| This Model is valid for Automotive grade 2 Temperature Range -40C<=Tc<=105C
| Valid for LPDDR4-4266 operation
| Part Number   VDD/VDDQ   Package   Architecture
| SCE11U48324AF-04ZA2   1.1 +0.07/-0.04  FBGA   1.5G bit x 32 (200b,QDP,10x14.5x1.1)
[IBIS Ver]  5.0
[File Name] usesnxx32aa2.ibs
[Date]   06/26/2025
[File Rev]  1.0
[Source] Simulation of a silicon level SPICE model
[Notes]  IBIS Characteristics for I/O Buffer
  IBIS Model Revision History: Rev 1.0:
  2025-06-26 - IBIS model file initial creation
[Disclaimer]  The IBIS models are for modeling purpose only and are subject to change without any notice. UniIC is not
  responsible for any problems the models may cause.
[Copyright] Copyright 2025 UniIC Semiconductors Corp. All rights reserved
|   Component SCE11U48324AF-04ZA2
[Component] SCE11U48324AF-04ZA2
[Manufacturer] UniIC Semiconductors Corp.
[Package]
|   typ   min   max
R_pkg   1377.8m   678.01m   2200.4m
L_pkg   2.871nH   1.351nH   4.718nH
C_pkg   1.060pF   0.653pF   1.525pF
[Pin] signal_name  model_name   R_pin   L_pin   C_pin
A1   DNU   NC
A2   DNU   NC
A3   VSS   GND
A4   VDD2   POWER
A5   ZQ0   NC
A8   ZQ1   NC
A9   VDD2   POWER
A10   VSS   GND
A11   DNU   NC
A12   DNU   NC
B1   DNU   NC
B2   DQ0_A   DQ   815.75m   1.783nH   0.708pF
B3   VDDQ   POWER
B4   DQ7_A   DQ   837.92m   1.787nH   0.739pF
B5   VDDQ   POWER
B8   VDDQ   POWER
B9   DQ15_A   DQ   841.56m   1.773nH   0.739pF
B10   VDDQ   POWER
B11   DQ8_A   DQ   884.91m   1.894nH   0.764pF
B12   DNU   NC
C1   VSS   GND
C2   DQ1_A   DQ   862.48m   1.799nH   0.724pF
C3   DMI0_A   DQ   832.58m   1.719nH   0.717pF
C4   DQ6_A   DQ   753.90m   1.588nH   0.689pF
C5   VSS   GND
C8   VSS   GND
C9   DQ14_A   DQ   814.61m   1.676nH   0.743pF
C10   DMI1_A   DQ   820.28m   1.690nH   0.736pF
C11   DQ9_A   DQ   853.94m   1.774nH   0.747pF
C12   VSS   GND
D1   VDDQ   POWER
D2   VSS   GND
D3   DQS0_t_A   DQS   780.62m   1.630nH   0.669pF
D4   VSS   GND
D5   VDDQ   POWER
D8   VDDQ   POWER
D9   VSS   GND
D10   DQS1_t_A   DQS   780.55m   1.628nH   0.668pF
D11   VSS   GND
D12   VDDQ   POWER
E1   VSS   GND
E2   DQ2_A   DQ   769.99m   1.582nH   0.719pF
E3   DQS0_c_A   DQS   796.22m   1.643nH   0.667pF
E4   DQ5_A   DQ   693.55m   1.405nH   0.687pF
E5   VSS   GND
E8   VSS   GND
E9   DQ13_A   DQ   692.33m   1.403nH   0.695pF
E10   DQS1_c_A   DQS   796.67m   1.642nH   0.671pF
E11   DQ10_A   DQ   751.10m   1.558nH   0.707pF
E12   VSS   GND
F1   VDD1   POWER
F2   DQ3_A   DQ   803.96m   1.656nH   0.728pF
F3   VDDQ   POWER
F4   DQ4_A   DQ   678.01m   1.373nH   0.653pF
F5   VDD2   POWER
F8   VDD2   POWER
F9   DQ12_A   DQ   678.86m   1.351nH   0.678pF
F10   VDDQ   POWER
F11   DQ11_A   DQ   777.70m   1.621nH   0.719pF
F12   VDD1   POWER
G1   VSS   GND
G2   NC   NC
G3   VSS   GND
G4   VDD1   POWER
G5   VSS   GND
G8   VSS   GND
G9   VDD1   POWER
G10   VSS   GND
G11   NC   NC
G12   VSS   GND
H1   VDD2   POWER
H2   CA0_A   CA_INPUT   1149.9m   2.416nH   0.957pF
H3   CS1_A   CS_INPUT
H4   CS0_A   CS_INPUT
H5   VDD2   POWER
H8   VDD2   POWER
H9   CA2_A   CA_INPUT   1114.3m   2.201nH   0.964pF
H10   CA3_A   CA_INPUT   1179.0m   2.324nH   1.007pF
H11   CA4_A   CA_INPUT   1281.5m   2.502nH   1.076pF
H12   VDD2   POWER
J1   VSS   GND
J2   CA1_A   CA_INPUT   1241.5m   2.547nH   1.026pF
J3   VSS   GND
J4   CKE0_A   CKE_INPUT
J5   CKE1_A   CKE_INPUT
J8   CK_t_A   CLK_INPUT   1164.4m   2.511nH   0.936pF
J9   CK_c_A   CLK_INPUT   1179.6m   2.532nH   0.945pF
J10   VSS   GND
J11   CA5_A   CA_INPUT   1353.8m   2.632nH   1.108pF
J12   VSS   GND
K1   VDD2   POWER
K2   VSS   GND
K3   VDD2   POWER
K4   VSS   GND
K5   NC   NC
K8   NC   NC
K9   VSS   GND
K10   VDD2   POWER
K11   VSS   GND
K12   VDD2   POWER
N1   VDD2   POWER
N2   VSS   GND
N3   VDD2   POWER
N4   VSS   GND
N5   NC   NC
N8   NC   NC
N9   VSS   GND
N10   VDD2   POWER
N11   VSS   GND
N12   VDD2   POWER
P1   VSS   GND
P2   CA1_B   CA_INPUT   1537.5m   3.379nH   1.134pF
P3   VSS   GND
P4   CKE0_B   CKE_INPUT
P5   CKE1_B   CKE_INPUT
P8   CK_t_B   CLK_INPUT   1530.3m   3.244nH   1.121pF
P9   CK_c_B   CLK_INPUT   1598.7m   3.371nH   1.166pF
P10   VSS   GND
P11   CA5_B   CA_INPUT   1748.8m   3.785nH   1.229pF
P12   VSS   GND
R1   VDD2   POWER
R2   CA0_B   CA_INPUT   1568.1m   3.442nH   1.146pF
R3   CS1_B   CS_INPUT
R4   CS0_B   CS_INPUT
R5   VDD2   POWER
R8   VDD2   POWER
R9   CA2_B   CA_INPUT   1529.7m   3.316nH   1.089pF
R10   CA3_B   CA_INPUT   1595.3m   3.372nH   1.142pF
R11   CA4_B   CA_INPUT   1737.9m   3.619nH   1.236pF
R12   VDD2   POWER
T1   VSS   GND
T2   NC   NC
T3   VSS   GND
T4   VDD1   POWER
T5   VSS   GND
T8   VSS   GND
T9   VDD1   POWER
T10   VSS   GND
T11   RESET_n   NC
T12   VSS   GND
U1   VDD1   POWER
U2   DQ3_B   DQ   1783.2m   3.716nH   1.313pF
U3   VDDQ   POWER
U4   DQ4_B   DQ   1690.1m   3.453nH   1.244pF
U5   VDD2   POWER
U8   VDD2   POWER
U9   DQ12_B   DQ   1997.2m   3.951nH   1.469pF
U10   VDDQ   POWER
U11   DQ11_B   DQ   2089.2m   4.305nH   1.506pF
U12   VDD1   POWER
V1   VSS   GND
V2   DQ2_B   DQ   1862.6m   3.936nH   1.329pF
V3   DQS0_c_B   DQS   1877.9m   4.033nH   1.335pF
V4   DQ5_B   DQ   1694.8m   3.459nH   1.250pF
V5   VSS   GND
V8   VSS   GND
V9   DQ13_B   DQ   1972.8m   3.803nH   1.473pF
V10   DQS1_c_B   DQS   2092.9m   4.378nH   1.478pF
V11   DQ10_B   DQ   2200.4m   4.718nH   1.525pF
V12   VSS   GND
W1   VDDQ   POWER
W2   VSS   GND
W3   DQS0_t_B   DQS   1860.3m   4.071nH   1.335pF
W4   VSS   GND
W5   VDDQ   POWER
W8   VDDQ   POWER
W9   VSS   GND
W10   DQS1_t_B   DQS   2120.7m   4.481nH   1.515pF
W11   VSS   GND
W12   VDDQ   POWER
Y1   VSS   GND
Y2   DQ1_B   DQ   2023.5m   4.328nH   1.424pF
Y3   DMI0_B   DQ   1786.4m   3.621nH   1.340pF
Y4   DQ6_B   DQ   1702.5m   3.534nH   1.251pF
Y5   VSS   GND
Y8   VSS   GND
Y9   DQ14_B   DQ   1982.9m   3.898nH   1.426pF
Y10   DMI1_B   DQ   2061.8m   4.157nH   1.462pF
Y11   DQ9_B   DQ   2177.0m   4.685nH   1.515pF
Y12   VSS   GND
AA1   DNU   NC
AA2   DQ0_B   DQ   2060.0m   4.290nH   1.449pF
AA3   VDDQ   POWER
AA4   DQ7_B   DQ   1733.2m   3.601nH   1.258pF
AA5   VDDQ   POWER
AA8   VDDQ   POWER
AA9   DQ15_B   DQ   1970.9m   3.988nH   1.397pF
AA10  VDDQ   POWER
AA11  DQ8_B   DQ   2099.3m   4.696nH   1.451pF
AA12  DNU   NC
AB1   DNU   NC
AB2   DNU   NC
AB3   VSS   GND
AB4   VDD2   POWER
AB5   VSS   GND
AB8   VSS   GND
AB9   VDD2   POWER
AB10  VSS   GND
AB11  DNU   NC
AB12  DNU   NC
[Diff Pin]  inv_pin  vdiff   tdelay_typ   tdelay_min   tdelay_max
D3   E3   0.120V   0.000s   NA   NA
W3   V3   0.120V   0.000s   NA   NA
D10   E10   0.120V   0.000s   NA   NA
W10   V10   0.120V   0.000s   NA   NA
J8   J9   0.145V   0.000s   NA   NA
P8   P9   0.145V   0.000s   NA   NA
|   Model Selector
[Model Selector] DQ
| Data I/O models
DQ_PD40_SOC-ODT40_VOH30_4266   40 Ohm Pulldown, 40 Ohm System ODT Setting, VOH=VDDQ/3.0, 3200-4266Mbps
DQ_PD40_SOC-ODT48_VOH30_4266   40 Ohm Pulldown, 48 Ohm System ODT Setting, VOH=VDDQ/3.0, 3200-4266Mbps
DQ_PD40_SOC-ODT60_VOH30_4266   40 Ohm Pulldown, 60 Ohm System ODT Setting, VOH=VDDQ/3.0, 3200-4266Mbps
DQ_PD40_SOC-ODT80_VOH30_4266   40 Ohm Pulldown, 80 Ohm System ODT Setting, VOH=VDDQ/3.0, 3200-4266Mbps
DQ_PD40_SOC-ODT120_VOH30_4266   40 Ohm Pulldown, 120 Ohm System ODT Setting, VOH=VDDQ/3.0, 3200-4266Mbps
DQ_PD40_SOC-ODT240_VOH30_4266   40 Ohm Pulldown, 240 Ohm System ODT Setting, VOH=VDDQ/3.0, 3200-4266Mbps
DQ_PD40_SOC-ODTDIS_VOH30_4266   40 Ohm Pulldown, SOC ODT disabled setting, VOH=VDDQ/3.0 cal. point, 3200-4266Mbps
DQ_PD40_SOC-ODT80_VOH25_4266   40 Ohm Pulldown, 80 Ohm System ODT Setting, VOH=VDDQ/2.5, 3200-4266Mbps
DQ_PD40_SOC-ODT120_VOH25_4266   40 Ohm Pulldown, 120 Ohm System ODT Setting, VOH=VDDQ/2.5, 3200-4266Mbps
DQ_PD40_SOC-ODT240_VOH25_4266   40 Ohm Pulldown, 240 Ohm System ODT Setting, VOH=VDDQ/2.5, 3200-4266Mbps
DQ_PD40_SOC-ODTDIS_VOH25_4266   40 Ohm Pulldown, SOC ODT disabled setting, VOH=VDDQ/2.5 cal. point, 3200-4266Mbps
DQ_PD48_SOC-ODT40_VOH30_4266   48 Ohm Pulldown, 40 Ohm System ODT Setting, VOH=VDDQ/3.0, 3200-4266Mbps
DQ_PD48_SOC-ODT48_VOH30_4266   48 Ohm Pulldown, 48 Ohm System ODT Setting, VOH=VDDQ/3.0, 3200-4266Mbps
DQ_PD48_SOC-ODT60_VOH30_4266   48 Ohm Pulldown, 60 Ohm System ODT Setting, VOH=VDDQ/3.0, 3200-4266Mbps
DQ_PD48_SOC-ODT80_VOH30_4266   48 Ohm Pulldown, 80 Ohm System ODT Setting, VOH=VDDQ/3.0, 3200-4266Mbps
DQ_PD48_SOC-ODT120_VOH30_4266   48 Ohm Pulldown, 120 Ohm System ODT Setting, VOH=VDDQ/3.0, 3200-4266Mbps
DQ_PD48_SOC-ODT240_VOH30_4266   48 Ohm Pulldown, 240 Ohm System ODT Setting, VOH=VDDQ/3.0, 3200-4266Mbps
DQ_PD48_SOC-ODTDIS_VOH30_4266   48 Ohm Pulldown, SOC ODT disabled setting, VOH=VDDQ/3.0 cal. point, 3200-4266Mbps
DQ_PD48_SOC-ODT80_VOH25_4266   48 Ohm Pulldown, 80 Ohm System ODT Setting, VOH=VDDQ/2.5, 3200-4266Mbps
DQ_PD48_SOC-ODT120_VOH25_4266   48 Ohm Pulldown, 120 Ohm System ODT Setting, VOH=VDDQ/2.5, 3200-4266Mbps
DQ_PD48_SOC-ODT240_VOH25_4266   48 Ohm Pulldown, 240 Ohm System ODT Setting, VOH=VDDQ/2.5, 3200-4266Mbps
DQ_PD48_SOC-ODTDIS_VOH25_4266   48 Ohm Pulldown, SOC ODT disabled setting, VOH=VDDQ/2.5 cal. point, 3200-4266Mbps
DQ_PD60_SOC-ODT40_VOH30_4266   60 Ohm Pulldown, 40 Ohm System ODT Setting, VOH=VDDQ/3.0, 3200-4266Mbps
DQ_PD60_SOC-ODT48_VOH30_4266   60 Ohm Pulldown, 48 Ohm System ODT Setting, VOH=VDDQ/3.0, 3200-4266Mbps
DQ_PD60_SOC-ODT60_VOH30_4266   60 Ohm Pulldown, 60 Ohm System ODT Setting, VOH=VDDQ/3.0, 3200-4266Mbps
DQ_PD60_SOC-ODT80_VOH30_4266   60 Ohm Pulldown, 80 Ohm System ODT Setting, VOH=VDDQ/3.0, 3200-4266Mbps
DQ_PD60_SOC-ODT120_VOH30_4266   60 Ohm Pulldown, 120 Ohm System ODT Setting, VOH=VDDQ/3.0, 3200-4266Mbps
DQ_PD60_SOC-ODT240_VOH30_4266   60 Ohm Pulldown, 240 Ohm System ODT Setting, VOH=VDDQ/3.0, 3200-4266Mbps
DQ_PD60_SOC-ODTDIS_VOH30_4266   60 Ohm Pulldown, SOC ODT disabled setting, VOH=VDDQ/3.0 cal. point, 3200-4266Mbps
DQ_PD60_SOC-ODT80_VOH25_4266   60 Ohm Pulldown, 80 Ohm System ODT Setting, VOH=VDDQ/2.5, 3200-4266Mbps
DQ_PD60_SOC-ODT120_VOH25_4266   60 Ohm Pulldown, 120 Ohm System ODT Setting, VOH=VDDQ/2.5, 3200-4266Mbps
DQ_PD60_SOC-ODT240_VOH25_4266   60 Ohm Pulldown, 240 Ohm System ODT Setting, VOH=VDDQ/2.5, 3200-4266Mbps
DQ_PD60_SOC-ODTDIS_VOH25_4266   60 Ohm Pulldown, SOC ODT disabled setting, VOH=VDDQ/2.5 cal. point, 3200-4266Mbps
DQ_PD80_SOC-ODT40_VOH30_4266   80 Ohm Pulldown, 40 Ohm System ODT Setting, VOH=VDDQ/3.0, 3200-4266Mbps
DQ_PD80_SOC-ODT48_VOH30_4266   80 Ohm Pulldown, 48 Ohm System ODT Setting, VOH=VDDQ/3.0, 3200-4266Mbps
DQ_PD80_SOC-ODT60_VOH30_4266   80 Ohm Pulldown, 60 Ohm System ODT Setting, VOH=VDDQ/3.0, 3200-4266Mbps
DQ_PD80_SOC-ODT80_VOH30_4266   80 Ohm Pulldown, 80 Ohm System ODT Setting, VOH=VDDQ/3.0, 3200-4266Mbps
DQ_PD80_SOC-ODT120_VOH30_4266   80 Ohm Pulldown, 120 Ohm System ODT Setting, VOH=VDDQ/3.0, 3200-4266Mbps
DQ_PD80_SOC-ODT240_VOH30_4266   80 Ohm Pulldown, 240 Ohm System ODT Setting, VOH=VDDQ/3.0, 3200-4266Mbps
DQ_PD80_SOC-ODTDIS_VOH30_4266   80 Ohm Pulldown, SOC ODT disabled setting, VOH=VDDQ/3.0 cal. point, 3200-4266Mbps
DQ_PD80_SOC-ODT80_VOH25_4266   80 Ohm Pulldown, 80 Ohm System ODT Setting, VOH=VDDQ/2.5, 3200-4266Mbps
DQ_PD80_SOC-ODT120_VOH25_4266   80 Ohm Pulldown, 120 Ohm System ODT Setting, VOH=VDDQ/2.5, 3200-4266Mbps
DQ_PD80_SOC-ODT240_VOH25_4266   80 Ohm Pulldown, 240 Ohm System ODT Setting, VOH=VDDQ/2.5, 3200-4266Mbps
DQ_PD80_SOC-ODTDIS_VOH25_4266   80 Ohm Pulldown, SOC ODT disabled setting, VOH=VDDQ/2.5 cal. point, 3200-4266Mbps
DQ_PD120_SOC-ODT40_VOH30_4266   120 Ohm Pulldown, 40 Ohm System ODT Setting, VOH=VDDQ/3.0, 3200-4266Mbps
DQ_PD120_SOC-ODT48_VOH30_4266   120 Ohm Pulldown, 48 Ohm System ODT Setting, VOH=VDDQ/3.0, 3200-4266Mbps
DQ_PD120_SOC-ODT60_VOH30_4266   120 Ohm Pulldown, 60 Ohm System ODT Setting, VOH=VDDQ/3.0, 3200-4266Mbps
DQ_PD120_SOC-ODT80_VOH30_4266   120 Ohm Pulldown, 80 Ohm System ODT Setting, VOH=VDDQ/3.0, 3200-4266Mbps
DQ_PD120_SOC-ODT120_VOH30_4266  120 Ohm Pulldown, 120 Ohm System ODT Setting, VOH=VDDQ/3.0, 3200-4266Mbps
DQ_PD120_SOC-ODT240_VOH30_4266  120 Ohm Pulldown, 240 Ohm System ODT Setting, VOH=VDDQ/3.0, 3200-4266Mbps
DQ_PD120_SOC-ODTDIS_VOH30_4266  120 Ohm Pulldown, SOC ODT disabled setting, VOH=VDDQ/3.0 cal. point, 3200-4266Mbps
DQ_PD120_SOC-ODT80_VOH25_4266   120 Ohm Pulldown, 80 Ohm System ODT Setting, VOH=VDDQ/2.5, 3200-4266Mbps
DQ_PD120_SOC-ODT120_VOH25_4266  120 Ohm Pulldown, 120 Ohm System ODT Setting, VOH=VDDQ/2.5, 3200-4266Mbps
DQ_PD120_SOC-ODT240_VOH25_4266  120 Ohm Pulldown, 240 Ohm System ODT Setting, VOH=VDDQ/2.5, 3200-4266Mbps
DQ_PD120_SOC-ODTDIS_VOH25_4266  120 Ohm Pulldown, SOC ODT disabled setting, VOH=VDDQ/2.5 cal. point, 3200-4266Mbps
DQ_PD240_SOC-ODT40_VOH30_4266   240 Ohm Pulldown, 40 Ohm System ODT Setting, VOH=VDDQ/3.0, 3200-4266Mbps
DQ_PD240_SOC-ODT48_VOH30_4266   240 Ohm Pulldown, 48 Ohm System ODT Setting, VOH=VDDQ/3.0, 3200-4266Mbps
DQ_PD240_SOC-ODT60_VOH30_4266   240 Ohm Pulldown, 60 Ohm System ODT Setting, VOH=VDDQ/3.0, 3200-4266Mbps
DQ_PD240_SOC-ODT80_VOH30_4266   240 Ohm Pulldown, 80 Ohm System ODT Setting, VOH=VDDQ/3.0, 3200-4266Mbps
DQ_PD240_SOC-ODT120_VOH30_4266  240 Ohm Pulldown, 120 Ohm System ODT Setting, VOH=VDDQ/3.0, 3200-4266Mbps
DQ_PD240_SOC-ODT240_VOH30_4266  240 Ohm Pulldown, 240 Ohm System ODT Setting, VOH=VDDQ/3.0, 3200-4266Mbps
DQ_PD240_SOC-ODTDIS_VOH30_4266  240 Ohm Pulldown, SOC ODT disabled setting, VOH=VDDQ/3.0 cal. point, 3200-4266Mbps
DQ_PD240_SOC-ODT80_VOH25_4266   240 Ohm Pulldown, 80 Ohm System ODT Setting, VOH=VDDQ/2.5, 3200-4266Mbps
DQ_PD240_SOC-ODT120_VOH25_4266  240 Ohm Pulldown, 120 Ohm System ODT Setting, VOH=VDDQ/2.5, 3200-4266Mbps
DQ_PD240_SOC-ODT240_VOH25_4266  240 Ohm Pulldown, 240 Ohm System ODT Setting, VOH=VDDQ/2.5, 3200-4266Mbps
DQ_PD240_SOC-ODTDIS_VOH25_4266  240 Ohm Pulldown, SOC ODT disabled setting, VOH=VDDQ/2.5 cal. point, 3200-4266Mbps
DQ_IN_ODTOFF_4266   with no ODT, 3200-4266Mbps
DQ_IN_ODT40_4266   with 40ohm ODT, 3200-4266Mbps
DQ_IN_ODT48_4266   with 48ohm ODT, 3200-4266Mbps
DQ_IN_ODT60_4266   with 60ohm ODT, 3200-4266Mbps
DQ_IN_ODT80_4266   with 80ohm ODT, 3200-4266Mbps
DQ_IN_ODT120_4266   with 120ohm ODT, 3200-4266Mbps
DQ_IN_ODT240_4266   with 240ohm ODT, 3200-4266Mbps
[Model Selector] DQS
| Data Strobe I/O models
DQS_PD40_SOC-ODT40_VOH30_4266   40 Ohm Pulldown, 40 Ohm System ODT Setting, VOH=VDDQ/3.0, 3200-4266Mbps
DQS_PD40_SOC-ODT48_VOH30_4266   40 Ohm Pulldown, 48 Ohm System ODT Setting, VOH=VDDQ/3.0, 3200-4266Mbps
DQS_PD40_SOC-ODT60_VOH30_4266   40 Ohm Pulldown, 60 Ohm System ODT Setting, VOH=VDDQ/3.0, 3200-4266Mbps
DQS_PD40_SOC-ODT80_VOH30_4266   40 Ohm Pulldown, 80 Ohm System ODT Setting, VOH=VDDQ/3.0, 3200-4266Mbps
DQS_PD40_SOC-ODT120_VOH30_4266  40 Ohm Pulldown, 120 Ohm System ODT Setting, VOH=VDDQ/3.0, 3200-4266Mbps
DQS_PD40_SOC-ODT240_VOH30_4266  40 Ohm Pulldown, 240 Ohm System ODT Setting, VOH=VDDQ/3.0, 3200-4266Mbps
DQS_PD40_SOC-ODTDIS_VOH30_4266  40 Ohm Pulldown, SOC ODT disabled setting, VOH=VDDQ/3.0 cal. point, 3200-4266Mbps
DQS_PD40_SOC-ODT80_VOH25_4266   40 Ohm Pulldown, 80 Ohm System ODT Setting, VOH=VDDQ/2.5, 3200-4266Mbps
DQS_PD40_SOC-ODT120_VOH25_4266  40 Ohm Pulldown, 120 Ohm System ODT Setting, VOH=VDDQ/2.5, 3200-4266Mbps
DQS_PD40_SOC-ODT240_VOH25_4266  40 Ohm Pulldown, 240 Ohm System ODT Setting, VOH=VDDQ/2.5, 3200-4266Mbps
DQS_PD40_SOC-ODTDIS_VOH25_4266  40 Ohm Pulldown, SOC ODT disabled setting, VOH=VDDQ/2.5 cal. point, 3200-4266Mbps
DQS_PD48_SOC-ODT40_VOH30_4266   48 Ohm Pulldown, 40 Ohm System ODT Setting, VOH=VDDQ/3.0, 3200-4266Mbps
DQS_PD48_SOC-ODT48_VOH30_4266   48 Ohm Pulldown, 48 Ohm System ODT Setting, VOH=VDDQ/3.0, 3200-4266Mbps
DQS_PD48_SOC-ODT60_VOH30_4266   48 Ohm Pulldown, 60 Ohm System ODT Setting, VOH=VDDQ/3.0, 3200-4266Mbps
DQS_PD48_SOC-ODT80_VOH30_4266   48 Ohm Pulldown, 80 Ohm System ODT Setting, VOH=VDDQ/3.0, 3200-4266Mbps
DQS_PD48_SOC-ODT120_VOH30_4266  48 Ohm Pulldown, 120 Ohm System ODT Setting, VOH=VDDQ/3.0, 3200-4266Mbps
DQS_PD48_SOC-ODT240_VOH30_4266  48 Ohm Pulldown, 240 Ohm System ODT Setting, VOH=VDDQ/3.0, 3200-4266Mbps
DQS_PD48_SOC-ODTDIS_VOH30_4266  48 Ohm Pulldown, SOC ODT disabled setting, VOH=VDDQ/3.0 cal. point, 3200-4266Mbps
DQS_PD48_SOC-ODT80_VOH25_4266   48 Ohm Pulldown, 80 Ohm System ODT Setting, VOH=VDDQ/2.5, 3200-4266Mbps
DQS_PD48_SOC-ODT120_VOH25_4266  48 Ohm Pulldown, 120 Ohm System ODT Setting, VOH=VDDQ/2.5, 3200-4266Mbps
DQS_PD48_SOC-ODT240_VOH25_4266  48 Ohm Pulldown, 240 Ohm System ODT Setting, VOH=VDDQ/2.5, 3200-4266Mbps
DQS_PD48_SOC-ODTDIS_VOH25_4266  48 Ohm Pulldown, SOC ODT disabled setting, VOH=VDDQ/2.5 cal. point, 3200-4266Mbps
DQS_PD60_SOC-ODT40_VOH30_4266   60 Ohm Pulldown, 40 Ohm System ODT Setting, VOH=VDDQ/3.0, 3200-4266Mbps
DQS_PD60_SOC-ODT48_VOH30_4266   60 Ohm Pulldown, 48 Ohm System ODT Setting, VOH=VDDQ/3.0, 3200-4266Mbps
DQS_PD60_SOC-ODT60_VOH30_4266   60 Ohm Pulldown, 60 Ohm System ODT Setting, VOH=VDDQ/3.0, 3200-4266Mbps
DQS_PD60_SOC-ODT80_VOH30_4266   60 Ohm Pulldown, 80 Ohm System ODT Setting, VOH=VDDQ/3.0, 3200-4266Mbps
DQS_PD60_SOC-ODT120_VOH30_4266  60 Ohm Pulldown, 120 Ohm System ODT Setting, VOH=VDDQ/3.0, 3200-4266Mbps
DQS_PD60_SOC-ODT240_VOH30_4266  60 Ohm Pulldown, 240 Ohm System ODT Setting, VOH=VDDQ/3.0, 3200-4266Mbps
DQS_PD60_SOC-ODTDIS_VOH30_4266  60 Ohm Pulldown, SOC ODT disabled setting, VOH=VDDQ/3.0 cal. point, 3200-4266Mbps
DQS_PD60_SOC-ODT80_VOH25_4266   60 Ohm Pulldown, 80 Ohm System ODT Setting, VOH=VDDQ/2.5, 3200-4266Mbps
DQS_PD60_SOC-ODT120_VOH25_4266  60 Ohm Pulldown, 120 Ohm System ODT Setting, VOH=VDDQ/2.5, 3200-4266Mbps
DQS_PD60_SOC-ODT240_VOH25_4266  60 Ohm Pulldown, 240 Ohm System ODT Setting, VOH=VDDQ/2.5, 3200-4266Mbps
DQS_PD60_SOC-ODTDIS_VOH25_4266  60 Ohm Pulldown, SOC ODT disabled setting, VOH=VDDQ/2.5 cal. point, 3200-4266Mbps
DQS_PD80_SOC-ODT40_VOH30_4266   80 Ohm Pulldown, 40 Ohm System ODT Setting, VOH=VDDQ/3.0, 3200-4266Mbps
DQS_PD80_SOC-ODT48_VOH30_4266   80 Ohm Pulldown, 48 Ohm System ODT Setting, VOH=VDDQ/3.0, 3200-4266Mbps
DQS_PD80_SOC-ODT60_VOH30_4266   80 Ohm Pulldown, 60 Ohm System ODT Setting, VOH=VDDQ/3.0, 3200-4266Mbps
DQS_PD80_SOC-ODT80_VOH30_4266   80 Ohm Pulldown, 80 Ohm System ODT Setting, VOH=VDDQ/3.0, 3200-4266Mbps
DQS_PD80_SOC-ODT120_VOH30_4266  80 Ohm Pulldown, 120 Ohm System ODT Setting, VOH=VDDQ/3.0, 3200-4266Mbps
DQS_PD80_SOC-ODT240_VOH30_4266  80 Ohm Pulldown, 240 Ohm System ODT Setting, VOH=VDDQ/3.0, 3200-4266Mbps
DQS_PD80_SOC-ODTDIS_VOH30_4266  80 Ohm Pulldown, SOC ODT disabled setting, VOH=VDDQ/3.0 cal. point, 3200-4266Mbps
DQS_PD80_SOC-ODT80_VOH25_4266   80 Ohm Pulldown, 80 Ohm System ODT Setting, VOH=VDDQ/2.5, 3200-4266Mbps
DQS_PD80_SOC-ODT120_VOH25_4266  80 Ohm Pulldown, 120 Ohm System ODT Setting, VOH=VDDQ/2.5, 3200-4266Mbps
DQS_PD80_SOC-ODT240_VOH25_4266  80 Ohm Pulldown, 240 Ohm System ODT Setting, VOH=VDDQ/2.5, 3200-4266Mbps
DQS_PD80_SOC-ODTDIS_VOH25_4266  80 Ohm Pulldown, SOC ODT disabled setting, VOH=VDDQ/2.5 cal. point, 3200-4266Mbps
DQS_PD120_SOC-ODT40_VOH30_4266  120 Ohm Pulldown, 40 Ohm System ODT Setting, VOH=VDDQ/3.0, 3200-4266Mbps
DQS_PD120_SOC-ODT48_VOH30_4266  120 Ohm Pulldown, 48 Ohm System ODT Setting, VOH=VDDQ/3.0, 3200-4266Mbps
DQS_PD120_SOC-ODT60_VOH30_4266  120 Ohm Pulldown, 60 Ohm System ODT Setting, VOH=VDDQ/3.0, 3200-4266Mbps
DQS_PD120_SOC-ODT80_VOH30_4266  120 Ohm Pulldown, 80 Ohm System ODT Setting, VOH=VDDQ/3.0, 3200-4266Mbps
DQS_PD120_SOC-ODT120_VOH30_4266 120 Ohm Pulldown, 120 Ohm System ODT Setting, VOH=VDDQ/3.0, 3200-4266Mbps
DQS_PD120_SOC-ODT240_VOH30_4266 120 Ohm Pulldown, 240 Ohm System ODT Setting, VOH=VDDQ/3.0, 3200-4266Mbps
DQS_PD120_SOC-ODTDIS_VOH30_4266 120 Ohm Pulldown, SOC ODT disabled setting, VOH=VDDQ/3.0 cal. point, 3200-4266Mbps
DQS_PD120_SOC-ODT80_VOH25_4266  120 Ohm Pulldown, 80 Ohm System ODT Setting, VOH=VDDQ/2.5, 3200-4266Mbps
DQS_PD120_SOC-ODT120_VOH25_4266 120 Ohm Pulldown, 120 Ohm System ODT Setting, VOH=VDDQ/2.5, 3200-4266Mbps
DQS_PD120_SOC-ODT240_VOH25_4266 120 Ohm Pulldown, 240 Ohm System ODT Setting, VOH=VDDQ/2.5, 3200-4266Mbps
DQS_PD120_SOC-ODTDIS_VOH25_4266 120 Ohm Pulldown, SOC ODT disabled setting, VOH=VDDQ/2.5 cal. point, 3200-4266Mbps
DQS_PD240_SOC-ODT40_VOH30_4266  240 Ohm Pulldown, 40 Ohm System ODT Setting, VOH=VDDQ/3.0, 3200-4266Mbps
DQS_PD240_SOC-ODT48_VOH30_4266  240 Ohm Pulldown, 48 Ohm System ODT Setting, VOH=VDDQ/3.0, 3200-4266Mbps
DQS_PD240_SOC-ODT60_VOH30_4266  240 Ohm Pulldown, 60 Ohm System ODT Setting, VOH=VDDQ/3.0, 3200-4266Mbps
DQS_PD240_SOC-ODT80_VOH30_4266  240 Ohm Pulldown, 80 Ohm System ODT Setting, VOH=VDDQ/3.0, 3200-4266Mbps
DQS_PD240_SOC-ODT120_VOH30_4266 240 Ohm Pulldown, 120 Ohm System ODT Setting, VOH=VDDQ/3.0, 3200-4266Mbps
DQS_PD240_SOC-ODT240_VOH30_4266 240 Ohm Pulldown, 240 Ohm System ODT Setting, VOH=VDDQ/3.0, 3200-4266Mbps
DQS_PD240_SOC-ODTDIS_VOH30_4266 240 Ohm Pulldown, SOC ODT disabled setting, VOH=VDDQ/3.0 cal. point, 3200-4266Mbps
DQS_PD240_SOC-ODT80_VOH25_4266  240 Ohm Pulldown, 80 Ohm System ODT Setting, VOH=VDDQ/2.5, 3200-4266Mbps
DQS_PD240_SOC-ODT120_VOH25_4266 240 Ohm Pulldown, 120 Ohm System ODT Setting, VOH=VDDQ/2.5, 3200-4266Mbps
DQS_PD240_SOC-ODT240_VOH25_4266 240 Ohm Pulldown, 240 Ohm System ODT Setting, VOH=VDDQ/2.5, 3200-4266Mbps
DQS_PD240_SOC-ODTDIS_VOH25_4266 240 Ohm Pulldown, SOC ODT disabled setting, VOH=VDDQ/2.5 cal. point, 3200-4266Mbps
DQS_IN_ODTOFF_4266   with no ODT, 3200-4266Mbps
DQS_IN_ODT40_4266   with 40ohm ODT, 3200-4266Mbps
DQS_IN_ODT48_4266   with 48ohm ODT, 3200-4266Mbps
DQS_IN_ODT60_4266   with 60ohm ODT, 3200-4266Mbps
DQS_IN_ODT80_4266   with 80ohm ODT, 3200-4266Mbps
DQS_IN_ODT120_4266   with 120ohm ODT, 3200-4266Mbps
DQS_IN_ODT240_4266   with 240ohm ODT, 3200-4266Mbps
[Model Selector] CA_INPUT
| CA Input models
CA_INPUT_ODTOFF_4266   with no ODT, 3200-4266Mbps
CA_INPUT_ODT40_4266   with 40ohm ODT, 3200-4266Mbps
CA_INPUT_ODT48_4266   with 48ohm ODT, 3200-4266Mbps
CA_INPUT_ODT60_4266   with 60ohm ODT, 3200-4266Mbps
CA_INPUT_ODT80_4266   with 80ohm ODT, 3200-4266Mbps
CA_INPUT_ODT120_4266   with 120ohm ODT, 3200-4266Mbps
CA_INPUT_ODT240_4266   with 240ohm ODT, 3200-4266Mbps
[Model Selector] CS_INPUT
| CS Input models
CS_INPUT_ODTOFF_4266   with no ODT, 3200-4266Mbps
CS_INPUT_ODT40_4266   with 40ohm ODT, 3200-4266Mbps
CS_INPUT_ODT48_4266   with 48ohm ODT, 3200-4266Mbps
CS_INPUT_ODT60_4266   with 60ohm ODT, 3200-4266Mbps
CS_INPUT_ODT80_4266   with 80ohm ODT, 3200-4266Mbps
CS_INPUT_ODT120_4266   with 120ohm ODT, 3200-4266Mbps
CS_INPUT_ODT240_4266   with 240ohm ODT, 3200-4266Mbps
[Model Selector] CLK_INPUT
| Clock Input models
CLK_INPUT_ODTOFF_4266   with no ODT, 3200-4266Mbps
CLK_INPUT_ODT40_4266   with 40ohm ODT, 3200-4266Mbps
CLK_INPUT_ODT48_4266   with 48ohm ODT, 3200-4266Mbps
CLK_INPUT_ODT60_4266   with 60ohm ODT, 3200-4266Mbps
CLK_INPUT_ODT80_4266   with 80ohm ODT, 3200-4266Mbps
CLK_INPUT_ODT120_4266   with 120ohm ODT, 3200-4266Mbps
CLK_INPUT_ODT240_4266   with 240ohm ODT, 3200-4266Mbps
| Models and submodels in the file (175): DQ_PD40_SOC-ODT40_VOH30_4266 (I/O), DQ_PD40_SOC-ODT48_VOH30_4266 (I/O), DQ_PD40_SOC-ODT60_VOH30_4266 (I/O), DQ_PD40_SOC-ODT80_VOH30_4266 (I/O), DQ_PD40_SOC-ODT120_VOH30_4266 (I/O), DQ_PD40_SOC-ODT240_VOH30_4266 (I/O), DQ_PD40_SOC-ODTDIS_VOH30_4266 (I/O), DQ_PD40_SOC-ODT80_VOH25_4266 (I/O), DQ_PD40_SOC-ODT120_VOH25_4266 (I/O), DQ_PD40_SOC-ODT240_VOH25_4266 (I/O), DQ_PD40_SOC-ODTDIS_VOH25_4266 (I/O), DQ_PD48_SOC-ODT40_VOH30_4266 (I/O), DQ_PD48_SOC-ODT48_VOH30_4266 (I/O), DQ_PD48_SOC-ODT60_VOH30_4266 (I/O), DQ_PD48_SOC-ODT80_VOH30_4266 (I/O), DQ_PD48_SOC-ODT120_VOH30_4266 (I/O), DQ_PD48_SOC-ODT240_VOH30_4266 (I/O), DQ_PD48_SOC-ODTDIS_VOH30_4266 (I/O), DQ_PD48_SOC-ODT80_VOH25_4266 (I/O), DQ_PD48_SOC-ODT120_VOH25_4266 (I/O), DQ_PD48_SOC-ODT240_VOH25_4266 (I/O), DQ_PD48_SOC-ODTDIS_VOH25_4266 (I/O), DQ_PD60_SOC-ODT40_VOH30_4266 (I/O), DQ_PD60_SOC-ODT48_VOH30_4266 (I/O), DQ_PD60_SOC-ODT60_VOH30_4266 (I/O), DQ_PD60_SOC-ODT80_VOH30_4266 (I/O), DQ_PD60_SOC-ODT120_VOH30_4266 (I/O), DQ_PD60_SOC-ODT240_VOH30_4266 (I/O), DQ_PD60_SOC-ODTDIS_VOH30_4266 (I/O), DQ_PD60_SOC-ODT80_VOH25_4266 (I/O), DQ_PD60_SOC-ODT120_VOH25_4266 (I/O), DQ_PD60_SOC-ODT240_VOH25_4266 (I/O), DQ_PD60_SOC-ODTDIS_VOH25_4266 (I/O), DQ_PD80_SOC-ODT40_VOH30_4266 (I/O), DQ_PD80_SOC-ODT48_VOH30_4266 (I/O), DQ_PD80_SOC-ODT60_VOH30_4266 (I/O), DQ_PD80_SOC-ODT80_VOH30_4266 (I/O), DQ_PD80_SOC-ODT120_VOH30_4266 (I/O), DQ_PD80_SOC-ODT240_VOH30_4266 (I/O), DQ_PD80_SOC-ODTDIS_VOH30_4266 (I/O), DQ_PD80_SOC-ODT80_VOH25_4266 (I/O), DQ_PD80_SOC-ODT120_VOH25_4266 (I/O), DQ_PD80_SOC-ODT240_VOH25_4266 (I/O), DQ_PD80_SOC-ODTDIS_VOH25_4266 (I/O), DQ_PD120_SOC-ODT40_VOH30_4266 (I/O), DQ_PD120_SOC-ODT48_VOH30_4266 (I/O), DQ_PD120_SOC-ODT60_VOH30_4266 (I/O), DQ_PD120_SOC-ODT80_VOH30_4266 (I/O), DQ_PD120_SOC-ODT120_VOH30_4266 (I/O), DQ_PD120_SOC-ODT240_VOH30_4266 (I/O), DQ_PD120_SOC-ODTDIS_VOH30_4266 (I/O), DQ_PD120_SOC-ODT80_VOH25_4266 (I/O), DQ_PD120_SOC-ODT120_VOH25_4266 (I/O), DQ_PD120_SOC-ODT240_VOH25_4266 (I/O), DQ_PD120_SOC-ODTDIS_VOH25_4266 (I/O), DQ_PD240_SOC-ODT40_VOH30_4266 (I/O), DQ_PD240_SOC-ODT48_VOH30_4266 (I/O), DQ_PD240_SOC-ODT60_VOH30_4266 (I/O), DQ_PD240_SOC-ODT80_VOH30_4266 (I/O), DQ_PD240_SOC-ODT120_VOH30_4266 (I/O), DQ_PD240_SOC-ODT240_VOH30_4266 (I/O), DQ_PD240_SOC-ODTDIS_VOH30_4266 (I/O), DQ_PD240_SOC-ODT80_VOH25_4266 (I/O), DQ_PD240_SOC-ODT120_VOH25_4266 (I/O), DQ_PD240_SOC-ODT240_VOH25_4266 (I/O), DQ_PD240_SOC-ODTDIS_VOH25_4266 (I/O), DQ_IN_ODTOFF_4266 (Input), DQ_IN_ODT40_4266 (Input), DQ_IN_ODT48_4266 (Input), DQ_IN_ODT60_4266 (Input), DQ_IN_ODT80_4266 (Input), DQ_IN_ODT120_4266 (Input), DQ_IN_ODT240_4266 (Input), DQS_PD40_SOC-ODT40_VOH30_4266 (I/O), DQS_PD40_SOC-ODT48_VOH30_4266 (I/O), DQS_PD40_SOC-ODT60_VOH30_4266 (I/O), DQS_PD40_SOC-ODT80_VOH30_4266 (I/O), DQS_PD40_SOC-ODT120_VOH30_4266 (I/O), DQS_PD40_SOC-ODT240_VOH30_4266 (I/O), DQS_PD40_SOC-ODTDIS_VOH30_4266 (I/O)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
